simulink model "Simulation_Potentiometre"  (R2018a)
settings: Solver=VariableStepAuto  StartTime=0.0  StopTime=10  RelTol=1e-3
undefined symbols (not defined in the file): sigbuilder_block
libraries: simulink x1

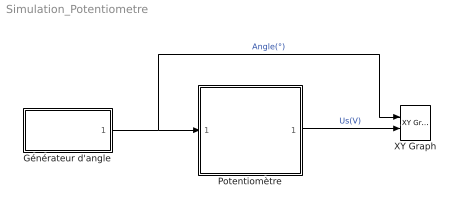
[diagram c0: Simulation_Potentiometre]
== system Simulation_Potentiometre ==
  Générateur d'angle : Subsystem  Tag=STV Subsys  LoadFcn=sigbuilder_block('load');  StartFcn=sigbuilder_block('start');  StopFcn=sigbuilder_block('stop');  ClipboardFcn=sigbuilder_block('clipboard');  mask(Sigbuilder block){tuvar=[0:10]}
      mask help: Simulink:masks:SigbuilderBlock_MD
      mask init:
      | if ~strcmp(get_param(bdroot(gcbh),'SimulationStatus'),'stopped') tuvar = sigbuilder_block('maskInit'); end
  Potentiomètre : Subsystem
  XY Graph : simulink/Sinks/XY Graph  xmin=-150  xmax=150  ymin=0  ymax=5  st=-1
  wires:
  Générateur d'angle/1(Angle) -> XY Graph/1, Potentiomètre/1(Angle)  "Angle(°)"
  Potentiomètre/1(Tension) -> XY Graph/2  "Us(V)"

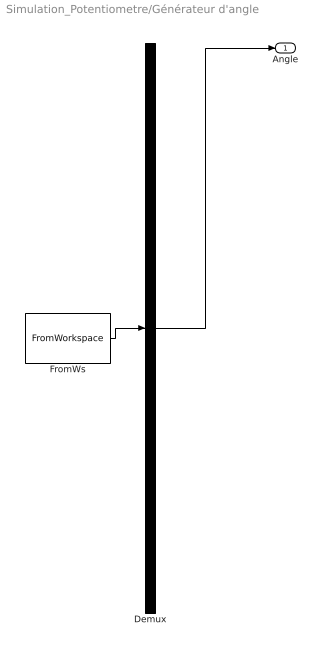
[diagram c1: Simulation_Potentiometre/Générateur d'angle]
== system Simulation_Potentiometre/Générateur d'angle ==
  Demux : Demux  Tag=STV Demux  Outputs=1
  FromWs : FromWorkspace  Tag=STV FromWs  VariableName=tuvar  SampleTime=0
  Angle : Outport  Tag=STV Outport
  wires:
  Demux/1 -> Angle/1
  FromWs/1 -> Demux/1

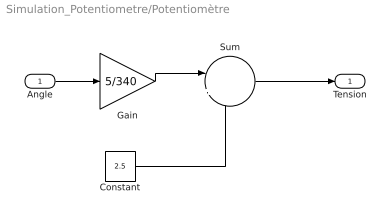
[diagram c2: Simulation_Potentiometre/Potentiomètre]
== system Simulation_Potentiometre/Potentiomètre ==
  Angle : Inport
  Constant : Constant  Value=2.5
  Gain : Gain  Gain=5/340
  Sum : Sum  Inputs=|++
  Tension : Outport
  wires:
  Constant/1 -> Sum/2
  Sum/1 -> Tension/1
  Angle/1 -> Gain/1
  Gain/1 -> Sum/1
